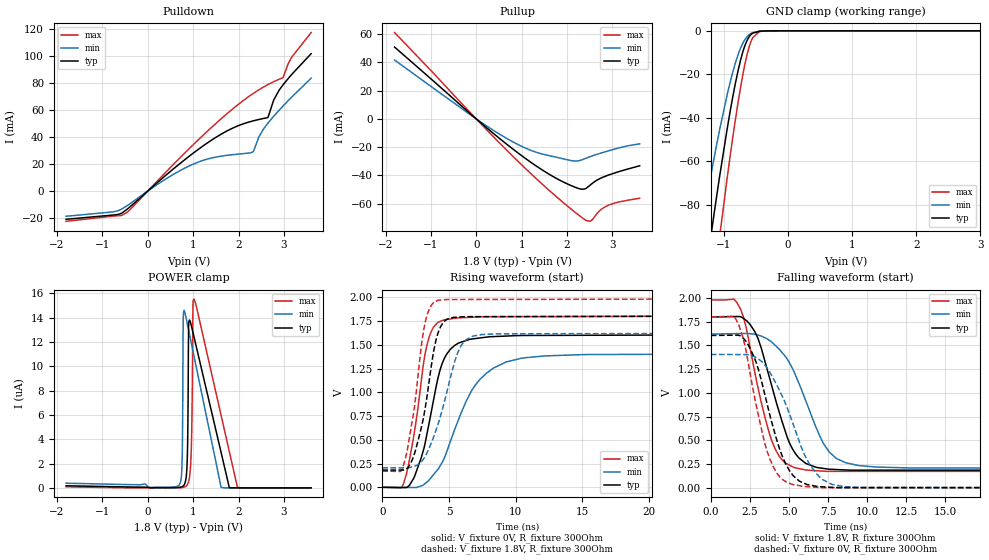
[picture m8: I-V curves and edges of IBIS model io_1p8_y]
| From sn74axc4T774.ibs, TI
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|   io_1p8_y Model
[Model]   io_1p8_y
Model_type   I/O
Polarity   Non-Inverting
Enable   Active-Low
Vinl = 0.63
Vinh = 1.17
Vmeas = 0.9
Vref = 0
Cref = 2pF
Rref = 100000
|   typ   min   max
C_comp   2.803pF   2.059pF   3.293pF
[Model spec]
|subparameter
Vinl   0.63   0.567   0.693
Vinh   1.17   1.053   1.287
| Where Nom  PVT is Nominal Process, 1.8V, 27C
|   Fast PVT is Strong Process,  1.98V, -40C
|   Slow PVT is Weak Process,   1.62V, 130C
[Voltage Range]   1.8   1.62   1.98
|Junction Temperature
[Temperature Range]   27   130   -40
[Pullup Reference]   1.8   1.62   1.98
[Pulldown Reference]   0   0   0
[Power Clamp Reference]   1.8   1.62   1.98
[GND Clamp Reference]   0   0   0
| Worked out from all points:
|   slope of the pulldown table from 0 to 0.27 V, typ, clamps not added: 33.8 ohm
|   slope of the pullup table from 0 to 0.27 V, typ, clamps not added: 36.5 ohm
|   GND clamp passes 1 mA (typ) near -0.54 V on its own axis
|   falling waveform, V_fixture 1.8V, R_fixture 300Ohm: 20-80 % time 1.74ns typ, 2.18ns min, 1.48ns max; typ from 1.8 V to 0.181 V
|   rising waveform, V_fixture 0V, R_fixture 300Ohm: 20-80 % time 1.51ns typ, 2.7ns min, 1.13ns max; typ from 0 V to 1.61 V
|   rising waveform, V_fixture 1.8V, R_fixture 300Ohm: 20-80 % time 1.21ns typ, 1.73ns min, 1.02ns max; typ from 0.181 V to 1.8 V
|   falling waveform, V_fixture 0V, R_fixture 300Ohm: 20-80 % time 1.63ns typ, 2.12ns min, 1.4ns max; typ from 1.61 V to 0 V
[Pulldown]
|   Voltage   I(typ)   I(min)   I(max)
-1.8V     -20.91mA   -18.68mA   -22.4mA
-757.8mV  -17.74mA   -15.41mA   -18.55mA
-444.6mV  -13.2mA    -10.62mA   -15.46mA
1.019V    28.48mA    20.16mA    34.85mA
1.748V    44.51mA    26.43mA    57.3mA
2.326V    51.96mA    29.07mA    72.25mA
2.444V    52.94mA    39.76mA    74.84mA
2.644V    54.39mA    50.14mA    78.72mA
2.774V    67.31mA    55.32mA    80.93mA
2.974V    78.29mA    62.67mA    83.86mA
3.173V    86.35mA    69.61mA    99.19mA
3.6V      101.7mA    83.51mA    117.3mA
[GND Clamp]
|   Voltage   I(typ)   I(min)   I(max)
-1.8V     -227.7mA   -173.3mA   -280.5mA
-1.314V   -118.5mA   -85.12mA   -156mA
-1.211V   -96.81mA   -68.22mA   -130.5mA
-1.114V   -76.99mA   -53.06mA   -106.8mA
-1.06V    -66.38mA   -45.06mA   -94mA
-898.2mV  -36.91mA   -23.54mA   -57.37mA
-774mV    -18.07mA   -10.82mA   -32.58mA
-671.4mV  -6.964mA   -4.128mA   -15.65mA
-574.2mV  -1.723mA   -1.197mA   -4.839mA
-444.6mV  -206.1uA   -178.2uA   -421.8uA
-342mV    -62.95uA   -50.11uA   -87.95uA
3.6V      0A         0A         0A
[Pullup]
|   Voltage   I(typ)   I(min)   I(max)
-1.8V     50.91mA    41.74mA    61.18mA
9mV       -250.5uA   -200.5uA   -303.9uA
840.6mV   -22.17mA   -16.84mA   -27.52mA
1.267V    -32.17mA   -23.03mA   -40.68mA
1.748V    -41.81mA   -27.01mA   -54.61mA
2.174V    -48.35mA   -29.83mA   -66.04mA
2.39V     -49.59mA   -28.2mA    -71.3mA
2.52V     -46.62mA   -26.58mA   -72.32mA
2.725V    -42.24mA   -24.4mA    -64.77mA
2.914V    -39.73mA   -22.59mA   -61.04mA
3.13V     -37.44mA   -20.62mA   -58.9mA
3.6V      -33.19mA   -17.66mA   -56.16mA
[POWER Clamp]
|   Voltage   I(typ)   I(min)   I(max)
-1.8V     171.8nA    383.4nA    88.28nA
689.4mV   39.1nA     223nA      575.5pA
754.2mV   97.12nA    1.895uA    18.8nA
781.2mV   159nA      14.01uA    37.55nA
867.6mV   2.112uA    13.55uA    243nA
900mV     13.42uA    12.97uA    522.5nA
959.4mV   13.35uA    11.9uA     3.252uA
997.2mV   12.76uA    11.22uA    15.28uA
1.013V    12.5uA     10.93uA    15.53uA
1.613V    2.958uA    63.04nA    6.012uA
1.975V    0A         0A         50.54nA
3.6V      0A         0A         0A
[Ramp]
R_load = 300
|   typ   min   max
dV/dt_r   0.96337/1.50058e-09   0.843144/2.68857e-09   1.08069/1.13026e-09
dV/dt_f   0.971137/1.73278e-09   0.849328/2.17439e-09   1.08576/1.469e-09
[Falling Waveform]
V_fixture = 1.8V
V_fixture_min = 1.62V
V_fixture_max = 1.98V
R_fixture = 300Ohm
C_fixture = 0F
|   Time   V(typ)   V(min)   V(max)
0s        1.8V       1.62V      1.98V
1.903ns   1.802V     1.626V     1.881V
3.02ns    1.572V     1.609V     1.052V
3.766ns   1.151V     1.551V     560.1mV
4.378ns   794.9mV    1.46V      332.2mV
5.605ns   319.9mV    1.111V     203.9mV
7.382ns   200.3mV    422.7mV    173.9mV
8.618ns   188.5mV    265mV      173.9mV
12.78ns   186.4mV    209.8mV    173.9mV
500ns     181.4mV    204.4mV    170.4mV
[Rising Waveform]
V_fixture = 0V
V_fixture_min = 0V
V_fixture_max = 0V
R_fixture = 300Ohm
C_fixture = 0F
|   Time   V(typ)   V(min)   V(max)
0s        140.1nV    884.4nV    89.78nV
1.596ns   -2.47mV    -1.047mV   40.58mV
2.274ns   76.81mV    -1.493mV   472.1mV
2.922ns   312.3mV    15.14mV    1.119V
3.81ns    894.9mV    128.1mV    1.679V
4.843ns   1.404V     379.7mV    1.767V
7.382ns   1.573V     1.144V     1.794V
10.43ns   1.597V     1.358V     1.796V
15.48ns   1.6V       1.397V     1.798V
500ns     1.606V     1.405V     1.801V
[Rising Waveform]
V_fixture = 1.8V
V_fixture_min = 1.62V
V_fixture_max = 1.98V
R_fixture = 300Ohm
C_fixture = 0F
|   Time   V(typ)   V(min)   V(max)
0s        181.4mV    204.4mV    170.4mV
1.443ns   182.1mV    205.2mV    175.1mV
2.168ns   264.7mV    212.4mV    635.4mV
2.983ns   664.8mV    277.1mV    1.548V
3.305ns   911.6mV    350mV      1.786V
4.045ns   1.56V      609.1mV    1.959V
4.855ns   1.768V     1.012V     1.976V
6.091ns   1.795V     1.526V     1.976V
8.653ns   1.796V     1.615V     1.977V
500ns     1.8V       1.62V      1.98V
[Falling Waveform]
|Gnd
V_fixture = 0V
V_fixture_min = 0V
V_fixture_max = 0V
R_fixture = 300Ohm
C_fixture = 0F
|   Time   V(typ)   V(min)   V(max)
0s        1.606V     1.405V     1.801V
1.759ns   1.609V     1.404V     1.727V
2.89ns    1.325V     1.372V     879.1mV
3.596ns   886.2mV    1.263V     387.1mV
4.204ns   509.6mV    1.087V     158.9mV
5.282ns   125.1mV    661.8mV    34.82mV
5.988ns   46.73mV    349mV      13.93mV
7.093ns   11.12mV    95.79mV    2.571mV
9.685ns   2.587mV    2.798mV    2.558mV
500ns     184.2nV    883.3nV    53.23nV
